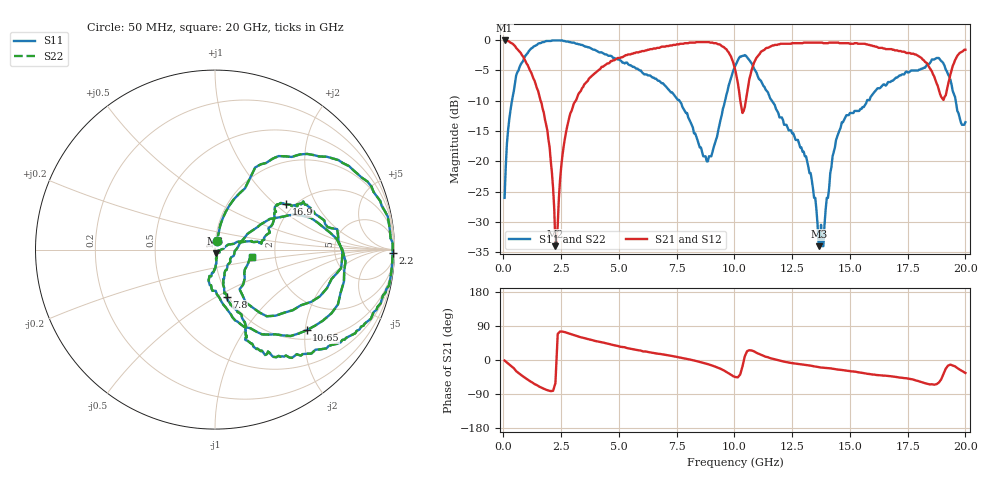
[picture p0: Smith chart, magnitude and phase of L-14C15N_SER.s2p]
#	mhz	s	ma	r	50
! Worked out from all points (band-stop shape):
!   400 points, 50 MHz to 20 GHz, reference 50 ohm
!   highest |S21| = -0.09 dB at 50 MHz (marker M1); lowest = -34.0 dB at 2.25 GHz (marker M2)
!   |S21| within 3 dB of the highest: 4.904 GHz to 9.886 GHz (4.982 GHz wide, 67.4 % of centre); 10.94 GHz to 18.12 GHz (7.188 GHz wide, 49.5 % of centre)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
!   lowest |S11| = -34.0 dB at 13.65 GHz (marker M3), VSWR 1.04, Z = 50.3 - j1.99 ohm
!   |S11| at or under -10 dB: 7.619 GHz to 9.594 GHz (1.975 GHz wide, 23 % of centre); 11.62 GHz to 15.74 GHz (4.122 GHz wide, 30.1 % of centre); 19.58 GHz to end of sweep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
!   |S22| runs from -34.0 to -0.1 dB; largest |S21 - S12| = 0
!   S11 on the Smith chart (normalised r, x): 50 MHz: 1.02, +0.10; 2.2 GHz: open; 7.8 GHz: 0.98, -0.56; 10.65 GHz: 1.22, -2.03; 16.9 GHz: 1.82, +1.18; 20 GHz: 1.51, -0.12
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50  0.05 77.0  0.99 -1.5  0.99 -1.5  0.05 77.0
550  0.51 63.9  0.86 -29.4  0.86 -29.4  0.51 63.9
1750  0.96 14.7  0.25 -76.0  0.25 -76.0  0.96 14.7
2200  0.99 -1.0  0.04 -71.0  0.04 -71.0  0.99 -1.0
2250  0.99 -2.9  0.02 -60.8  0.02 -60.8  0.99 -2.9
2650  0.98 -14.1  0.15 73.7  0.15 73.7  0.98 -14.1
3400  0.91 -30.8  0.4 59.3  0.4 59.3  0.91 -30.8
6700  0.46 -68.4  0.86 16.6  0.86 16.6  0.46 -68.4
7800  0.27 -75.9  0.93 4.7  0.93 4.7  0.27 -75.9
8850  0.1 -25.9  0.96 -10.7  0.96 -10.7  0.1 -25.9
10050  0.62 11.3  0.55 -45.1  0.55 -45.1  0.62 11.3
10350  0.74 -13.9  0.25 -16.7  0.25 -16.7  0.74 -13.9
10650  0.68 -41.4  0.48 25.8  0.48 25.8  0.68 -41.4
11650  0.31 -81.4  0.9 3.3  0.9 3.3  0.31 -81.4
13350  0.07 -83.4  0.95 -15.6  0.95 -15.6  0.07 -83.4
13650  0.02 -80.6  0.95 -18.8  0.95 -18.8  0.02 -80.6
14650  0.21 13.1  0.94 -26.4  0.94 -26.4  0.21 13.1
16700  0.45 35.0  0.84 -42.3  0.84 -42.3  0.45 35.0
16900  0.47 32.5  0.83 -43.9  0.83 -43.9  0.47 32.5
18750  0.71 -0.8  0.44 -63.9  0.44 -63.9  0.71 -0.8
19350  0.47 -52.2  0.52 -12.1  0.52 -12.1  0.47 -52.2
20000  0.21 -10.6  0.83 -34.2  0.83 -34.2  0.21 -10.6
